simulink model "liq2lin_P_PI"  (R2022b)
settings: Solver=ode45  StartTime=0.0  StopTime=60*10  FixedStep=1  RelTol=1e-6  EnableMultiTasking=on
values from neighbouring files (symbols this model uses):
  a = k12/(2*Ar*sqrt(h1b-h2b))    [para2Kp.m]    (also in nyqlog.m = log(spiralfactor)*2/pi)
  Ar = 6*25.4    (= 152.4)    [para2Kp.m]
  b = k2/(2*Ar*sqrt(h2b))    [para2Kp.m]
  h2b = (qb/k2)^2    (= 5.00000710049)    [para2Kp.m]
  k1 = 0    [para2Kp.m]
  k12 = 38    [para2Kp.m]
  k2 = 11.5    [para2Kp.m]
  Kp = 10    [para2Kp.m]
  qb = 25.7148    [para2Kp.m]
  qmax = 90    [para2Kp.m]
  qmin = -85    [para2Kp.m]
undefined symbols (not defined in the file or in its folder): Ki
libraries: simulink x1

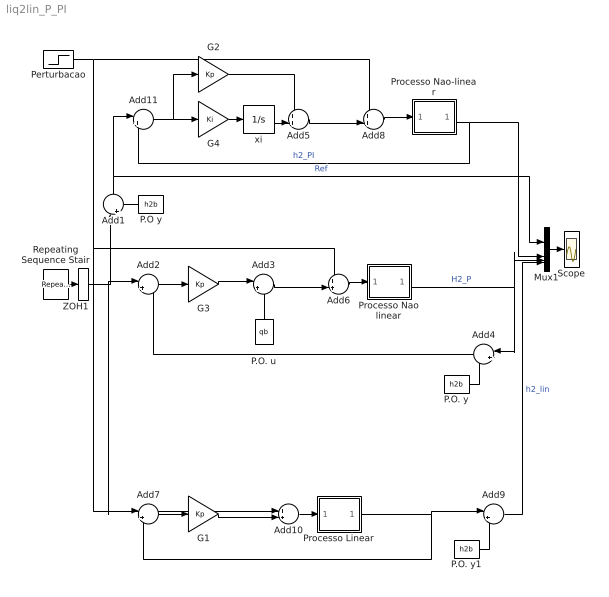
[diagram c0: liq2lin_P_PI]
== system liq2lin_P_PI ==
  Add1 : Sum  Inputs=|++
  Add{5..6,8,10} (4 alike) : Sum  Inputs=++|
  Add{2,4,7,11} (4 alike) : Sum  Inputs=|+-
  Add3 : Sum  Inputs=|++
  Add9 : Sum  Inputs=|++
  G1 : Gain  Gain=Kp
  G2 : Gain  Gain=Kp
  G3 : Gain  Gain=Kp
  G4 : Gain  Gain=Ki
  Mux1 : Mux
  P.O y : Constant  Value=h2b
  P.O. u : Constant  Value=qb
  P.O. y : Constant  Value=h2b
  P.O. y1 : Constant  Value=h2b
  Perturbacao : Step  Time=500  After=10  SampleTime=0
  Processo Nao-linear : Subsystem
  Processo Linear : Subsystem
  Processo Nao linear : Subsystem
  Repeating Sequence Stair : simulink/Sources/Repeating Sequence Stair  OutValues=[2 5 12 5 2].'-h2b  tsamp=100  OutMin=[]  OutMax=[]  OutDataTypeStr=double  OutputDataTypeScalingMode=double  OutDataType=fixdt(0,8)  ConRadixGroup=Best Precision: Vector-wise  OutScaling=2^-12
  Scope : Scope
  ZOH1 : ZeroOrderHold
  xi : Integrator
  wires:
  Mux1/1 -> Scope/1
  Add2/1 -> G3/1
  Processo Nao linear/2(H2) -> Mux1/3, Add4/1  "H2_P"
  P.O. u/1 -> Add3/2
  P.O y/1 -> Add1/2
  P.O. y/1 -> Add4/2
  Repeating Sequence Stair/1 -> ZOH1/1
  Add6/1 -> Processo Nao linear/1(u)
  Add3/1 -> Add6/2
  G3/1 -> Add3/1
  Add4/1 -> Add2/2
  Add7/1 -> G1/1
  P.O. y1/1 -> Add9/2
  Perturbacao/1 -> Add8/1, Add6/1, Add10/1
  Add10/1 -> Processo Linear/1(ul)
  Processo Linear/1(h2) -> Add9/1, Add7/2
  G1/1 -> Add10/2
  Add9/1 -> Mux1/4  "h2_lin"
  Add8/1 -> Processo Nao-linear/1(u)
  ZOH1/1 -> Add2/1, Add1/1, Add7/1
  Add5/1 -> Add8/2
  Processo Nao-linear/2(H2) -> Add11/2, Mux1/2  "h2_PI"
  xi/1 -> Add5/2
  G2/1 -> Add5/1
  Add11/1 -> G4/1, G2/1
  G4/1 -> xi/1
  Add1/1 -> Mux1/1, Add11/1  "Ref"

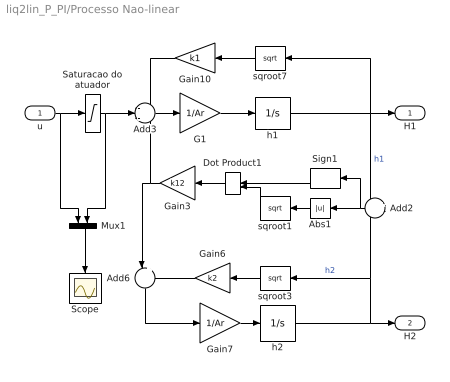
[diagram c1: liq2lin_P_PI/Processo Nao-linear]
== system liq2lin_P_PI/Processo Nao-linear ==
  u : Inport
  Abs1 : Abs
  Add2 : Sum  Inputs=+-
  Add3 : Sum  Inputs=-+-
  Add6 : Sum  Inputs=|+-
  Dot Product1 : DotProduct
  G1 : Gain  Gain=1/Ar
  Gain10 : Gain  Gain=k1
  Gain3 : Gain  Gain=k12
  Gain6 : Gain  Gain=k2
  Gain7 : Gain  Gain=1/Ar
  Mux1 : Mux  Inputs=2
  Saturacao do atuador : Saturate  UpperLimit=qmax  LowerLimit=qmin
  Scope : Scope
  Sign1 : Signum
  h1 : Integrator  LimitOutput=on  UpperSaturationLimit=16.5  LowerSaturationLimit=0
  h2 : Integrator  LimitOutput=on  UpperSaturationLimit=16.5  LowerSaturationLimit=0
  sqroot1 : Math  Operator=sqrt  SignedPower=on
  sqroot3 : Math  Operator=sqrt  SignedPower=on
  sqroot7 : Math  Operator=sqrt  SignedPower=on
  H1 : Outport
  H2 : Outport  Port=2
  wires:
  h1/1 -> Add2/1, H1/1, sqroot7/1  "h1"
  h2/1 -> Add2/2, sqroot3/1, H2/1  "h2"
  Saturacao do atuador/1 -> Add3/2, Mux1/2
  Add6/1 -> Gain7/1
  Gain10/1 -> Add3/1
  sqroot7/1 -> Gain10/1
  Gain6/1 -> Add6/2
  Gain7/1 -> h2/1
  sqroot3/1 -> Gain6/1
  G1/1 -> h1/1
  Gain3/1 -> Add6/1, Add3/3
  Add3/1 -> G1/1
  Dot Product1/1 -> Gain3/1
  sqroot1/1 -> Dot Product1/2
  Sign1/1 -> Dot Product1/1
  Abs1/1 -> sqroot1/1
  Add2/1 -> Abs1/1, Sign1/1
  u/1 -> Saturacao do atuador/1, Mux1/1
  Mux1/1 -> Scope/1

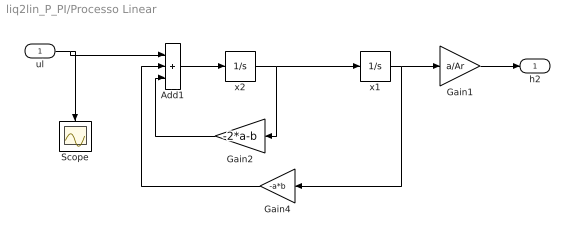
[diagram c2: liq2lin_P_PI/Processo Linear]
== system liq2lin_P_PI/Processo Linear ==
  ul : Inport
  Add1 : Sum  Inputs=+++
  Gain1 : Gain  Gain=a/Ar
  Gain2 : Gain  Gain=-2*a-b
  Gain4 : Gain  Gain=-a*b
  Scope : Scope
  x1 : Integrator
  x2 : Integrator
  h2 : Outport  VectorParamsAs1DForOutWhenUnconnected=off
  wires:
  ul/1 -> Scope/1, Add1/1
  x1/1 -> Gain4/1, Gain1/1
  x2/1 -> Gain2/1, x1/1
  Gain1/1 -> h2/1
  Add1/1 -> x2/1
  Gain2/1 -> Add1/3
  Gain4/1 -> Add1/2

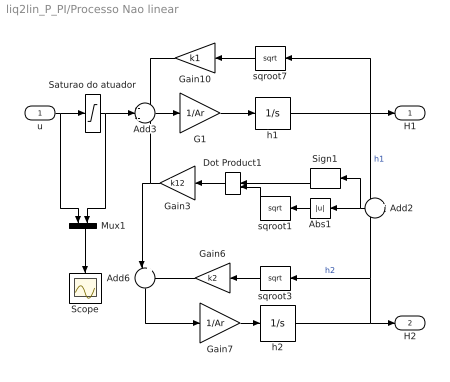
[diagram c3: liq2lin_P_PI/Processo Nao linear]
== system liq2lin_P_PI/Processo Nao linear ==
  u : Inport
  Abs1 : Abs
  Add2 : Sum  Inputs=+-
  Add3 : Sum  Inputs=-+-
  Add6 : Sum  Inputs=|+-
  Dot Product1 : DotProduct
  G1 : Gain  Gain=1/Ar
  Gain10 : Gain  Gain=k1
  Gain3 : Gain  Gain=k12
  Gain6 : Gain  Gain=k2
  Gain7 : Gain  Gain=1/Ar
  Mux1 : Mux  Inputs=2
  Saturao do atuador : Saturate  UpperLimit=qmax  LowerLimit=qmin
  Scope : Scope
  Sign1 : Signum
  h1 : Integrator  LimitOutput=on  UpperSaturationLimit=16.5  LowerSaturationLimit=0
  h2 : Integrator  LimitOutput=on  UpperSaturationLimit=16.5  LowerSaturationLimit=0
  sqroot1 : Math  Operator=sqrt  SignedPower=on
  sqroot3 : Math  Operator=sqrt  SignedPower=on
  sqroot7 : Math  Operator=sqrt  SignedPower=on
  H1 : Outport  VectorParamsAs1DForOutWhenUnconnected=off
  H2 : Outport  Port=2  VectorParamsAs1DForOutWhenUnconnected=off
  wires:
  h1/1 -> Add2/1, H1/1, sqroot7/1  "h1"
  h2/1 -> Add2/2, sqroot3/1, H2/1  "h2"
  Saturao do atuador/1 -> Add3/2, Mux1/2
  Add6/1 -> Gain7/1
  Gain10/1 -> Add3/1
  sqroot7/1 -> Gain10/1
  Gain6/1 -> Add6/2
  Gain7/1 -> h2/1
  sqroot3/1 -> Gain6/1
  G1/1 -> h1/1
  Gain3/1 -> Add6/1, Add3/3
  Add3/1 -> G1/1
  Dot Product1/1 -> Gain3/1
  sqroot1/1 -> Dot Product1/2
  Sign1/1 -> Dot Product1/1
  Abs1/1 -> sqroot1/1
  Add2/1 -> Abs1/1, Sign1/1
  u/1 -> Saturao do atuador/1, Mux1/1
  Mux1/1 -> Scope/1
